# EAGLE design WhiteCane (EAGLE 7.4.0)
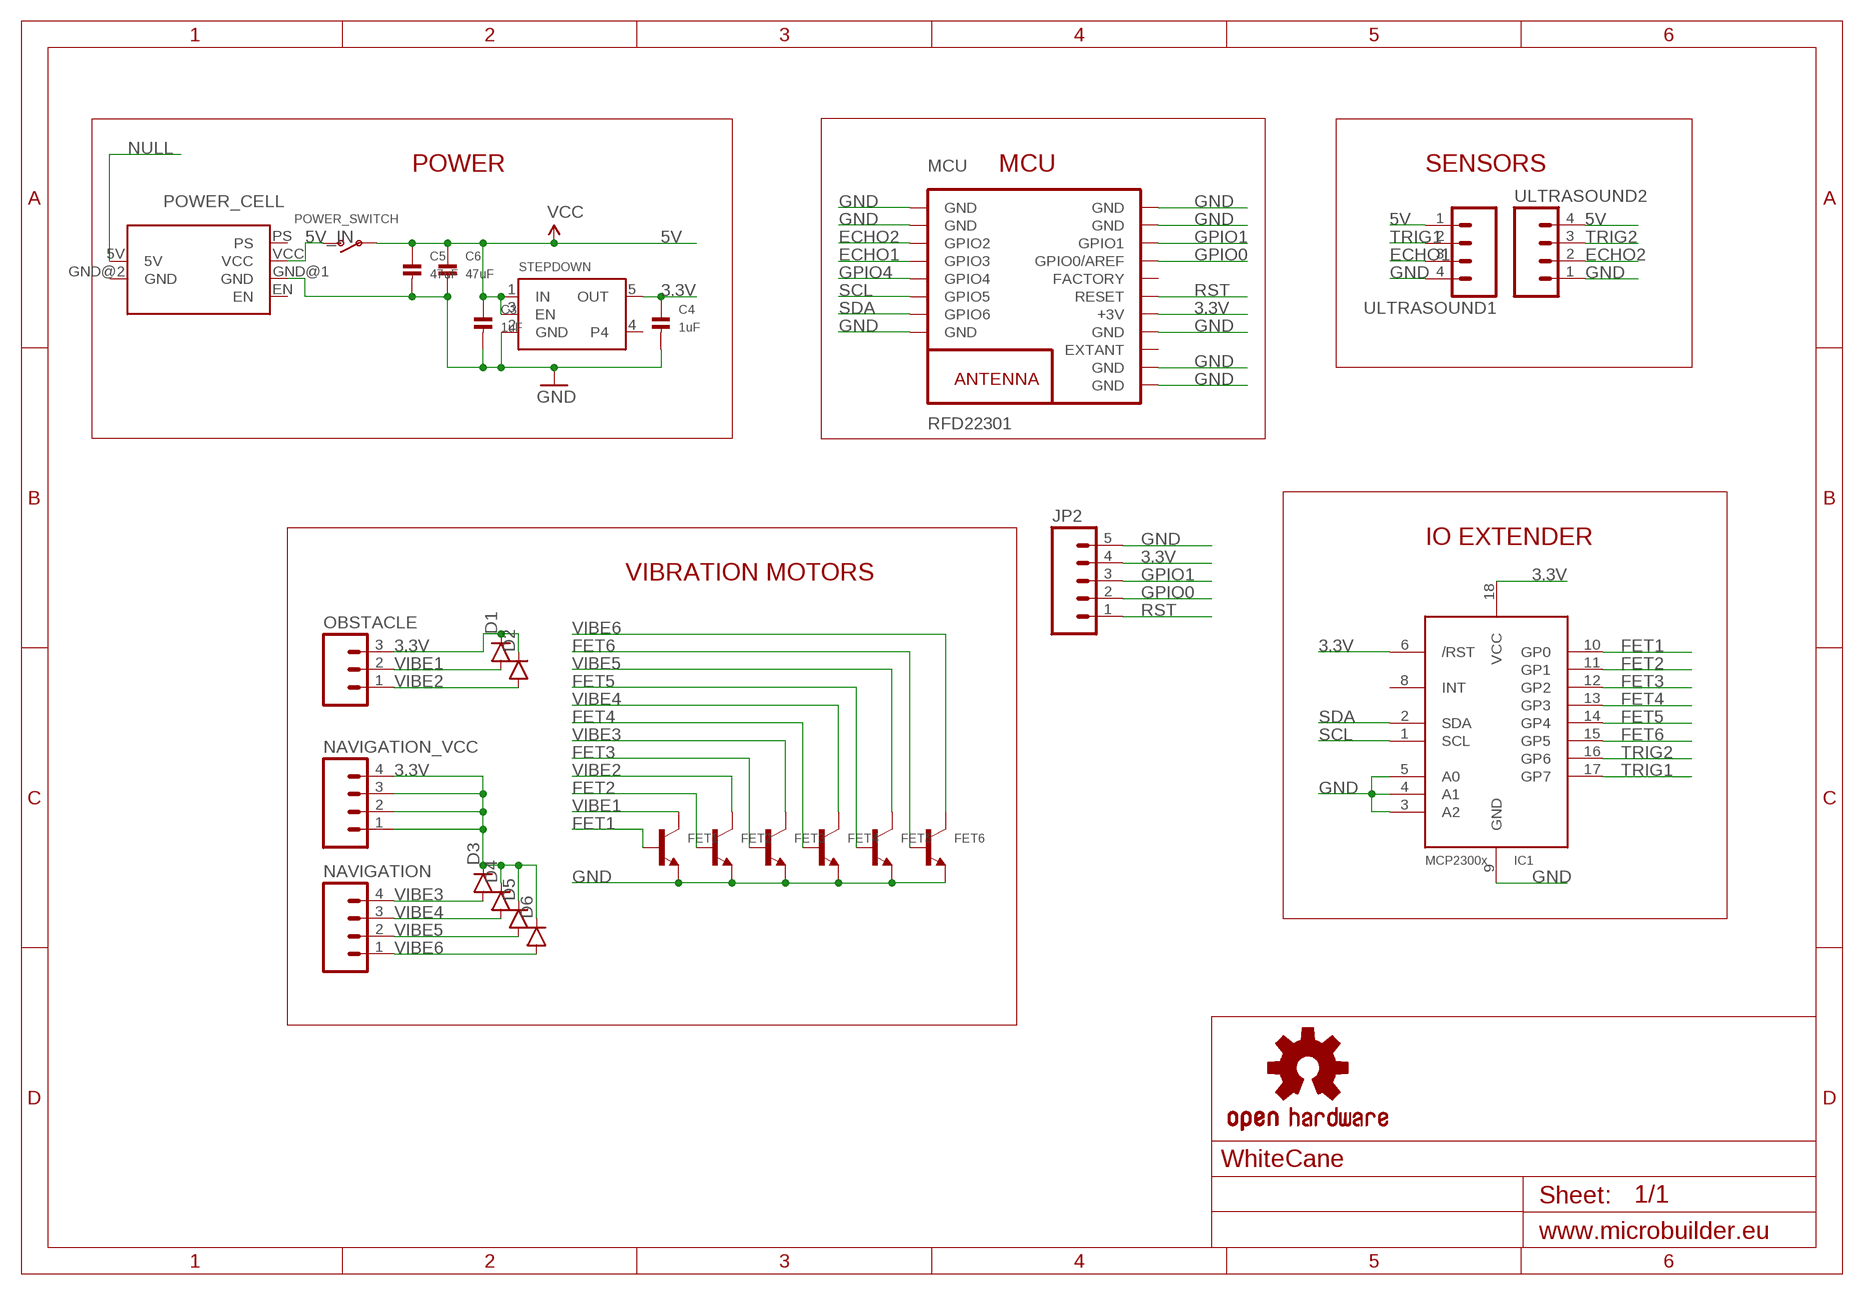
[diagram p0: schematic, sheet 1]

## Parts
C3  1uF  CAP_CERAMIC0603  [0603]
C4  1uF  CAP_CERAMIC0603  [0603]
C5  47uF  CAP_CERAMIC0805  [0805]
C6  47uF  CAP_CERAMIC0805  [0805]
D1  DIODESOD123  [SOD-123]
D2  DIODESOD123  [SOD-123]
D3  DIODESOD123  [SOD-123]
D4  DIODESOD123  [SOD-123]
D5  DIODESOD123  [SOD-123]
D6  DIODESOD123  [SOD-123]
FET1  TRANSISTOR_NPN  [SOT23-R]
FET2  TRANSISTOR_NPN  [SOT23-R]
FET3  TRANSISTOR_NPN  [SOT23-R]
FET4  TRANSISTOR_NPN  [SOT23-R]
FET5  TRANSISTOR_NPN  [SOT23-R]
FET6  TRANSISTOR_NPN  [SOT23-R]
IC1  MCP23008/SO  [SO18W]
JP2  M05PTH  [1X05]
MCU  RFD22301  [RFD22301]
NAVIGATION  M04PTH  [1X04]
NAVIGATION_VCC  M04PTH  [1X04]
OBSTACLE  M03PTH  [1X03]
POWER_CELL  POWER_CELL  [POWER_CELL]
POWER_SWITCH  SWITCH_SPST  [SPST_SMT_19192]
STEPDOWN  VREG_SOT23-5  [SOT23-5]
U$1  OSHW-LOGOS  [OSHW-LOGO-S]
ULTRASOUND1  M04PTH  [1X04]
ULTRASOUND2  M04PTH  [1X04]

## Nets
3.3V: C4.1 D1.C D2.C D3.C D4.C D5.C D6.C IC1.6(/RST) IC1.18(VCC) JP2.4 MCU.13(+3V) NAVIGATION_VCC.1 NAVIGATION_VCC.2 NAVIGATION_VCC.3 OBSTACLE.3 STEPDOWN.5(OUT)
5V: C3.1 C5.1 C6.1 POWER_SWITCH.B(P) STEPDOWN.1(IN) STEPDOWN.3(EN) ULTRASOUND1.1 ULTRASOUND2.4 ; supply symbol labelled VCC
5V_IN: POWER_CELL.VCC POWER_SWITCH.C(S)
ECHO1: MCU.4(GPIO3) ULTRASOUND1.3
ECHO2: MCU.3(GPIO2) ULTRASOUND2.2
FET1: FET1.1(B) IC1.10(GP0)
FET2: FET2.1(B) IC1.11(GP1)
FET3: FET3.1(B) IC1.12(GP2)
FET4: FET4.1(B) IC1.13(GP3)
FET5: FET5.1(B) IC1.14(GP4)
FET6: FET6.1(B) IC1.15(GP5)
GND: C3.2 C4.2 C5.2 C6.2 FET1.2(E) FET2.2(E) FET3.2(E) FET4.2(E) FET5.2(E) FET6.2(E) IC1.3(A2) IC1.4(A1) IC1.5(A0) IC1.9(GND) JP2.5 MCU.1(GND) MCU.2(GND) MCU.8(GND) MCU.9(GND) MCU.10(GND) MCU.12(GND) MCU.18(GND) MCU.19(GND) POWER_CELL.GND@1(GND) STEPDOWN.2(GND) ULTRASOUND1.4 ULTRASOUND2.1
GPIO0: JP2.2 MCU.16(GPIO0/AREF)
GPIO1: JP2.3 MCU.17(GPIO1)
GPIO4: MCU.5(GPIO4)
NULL: POWER_CELL.5V
RST: JP2.1 MCU.14(RESET)
SCL: IC1.1(SCL) MCU.6(GPIO5)
SDA: IC1.2(SDA) MCU.7(GPIO6)
TRIG1: IC1.17(GP7) ULTRASOUND1.2
TRIG2: IC1.16(GP6) ULTRASOUND2.3
VIBE1: D1.A FET1.3(C) OBSTACLE.2
VIBE2: D2.A FET2.3(C) OBSTACLE.1
VIBE3: D3.A FET3.3(C) NAVIGATION.4
VIBE4: D4.A FET4.3(C) NAVIGATION.3
VIBE5: D5.A FET5.3(C) NAVIGATION.2
VIBE6: D6.A FET6.3(C) NAVIGATION.1
Unconnected: IC1.8(INT) MCU.11(EXTANT) MCU.15(FACTORY) NAVIGATION_VCC.4 POWER_CELL.EN POWER_CELL.PS STEPDOWN.4

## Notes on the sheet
- POWER | MCU | SENSORS
- IO EXTENDER
- VIBRATION MOTORS

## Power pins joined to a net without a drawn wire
GND: POWER_CELL.GND@2(GND)

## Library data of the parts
C3-C6 = microbuilder:CAP_CERAMIC: Ceramic Capacitors
D1-D6 = SparkFun-DiscreteSemi:DIODE: Diode
FET1-FET6 = microbuilder:TRANSISTOR_NPN: NPN Transistor Transistor (NPN) 500mA 45V - BC817 [Digikey: 568-1631-1-ND] Transistor (NPN) 500mA 45V - BC817,215 [Mouser: 771-BC817-T/R] SOT23-R - SOT23 footprint optimised for use with solder paste and reflow ovens. SOT23-W - SOT23 footprint optimised for hand-soldering (larger pads).
IC1 = adafruit:MCP23008: MCP23008 Inexpensive i2c i/o expander - 8 general purpose i/o pins with optional pullups
JP2 = SparkFun-Connectors:M05: Header 5 Standard 5-pin 0.1" header. Use with straight break away headers (SKU : PRT-00116), right angle break away headers (PRT-00553), swiss pins (PRT-00743), machine pins (PRT-00117), and female headers (PRT-00115). Molex polarized connector foot print use with SKU : PRT-08230 with associated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
MCU = RF_Digital_RFD22301_Eagle_Schematic_PCB_Library:RFD22301: RFD22301 RFduino SMT Module RFD22301 Datasheet: http://www.rfdigital.com/wp-content/uploads/2014/03/RFD22301.Data_.Sheet_.11.24.13_11.38PM.pdf
NAVIGATION NAVIGATION_VCC ULTRASOUND1 ULTRASOUND2 = SparkFun-Connectors:M04: Header 4 Standard 4-pin 0.1" header. Use with straight break away headers (SKU : PRT-00116), right angle break away headers (PRT-00553), swiss pins (PRT-00743), machine pins (PRT-00117), and female headers (PRT-00115). Molex polarized connector foot print use with SKU : PRT-08231 with associated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
OBSTACLE = SparkFun-Connectors:M03: Header 3 Standard 3-pin 0.1" header. Use with straight break away headers (SKU : PRT-00116), right angle break away headers (PRT-00553), swiss pins (PRT-00743), machine pins (PRT-00117), and female headers (PRT-00115). Molex polarized connector foot print use with SKU : PRT-08232 with associated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
POWER_CELL = myParts:POWER_CELL
POWER_SWITCH = microbuilder:SWITCH_SPST: Switch - SPST
STEPDOWN = microbuilder:VREG_SOT23-5: SOT23-5 Fixed Voltage Regulators To better organise some of the SOT23-5 fixed voltage regulators in this library, this new part was created. Part Current Out V Out V In V Dropout Digikey Part No. ADP121 150mA 3.3V 3.4-5.5V 0.09V @ 150mA ADP121-AUJZ33R7CT-ND ADP121 150mA 3.0V 3.1-5.5V 0.09V @ 150mA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
U$1 = SparkFun:OSHW-LOGO: Open Source Hardware Logo This logo indicates the piece of hardware it is found on incorporates a OSHW license and/or adheres to the definition of open source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

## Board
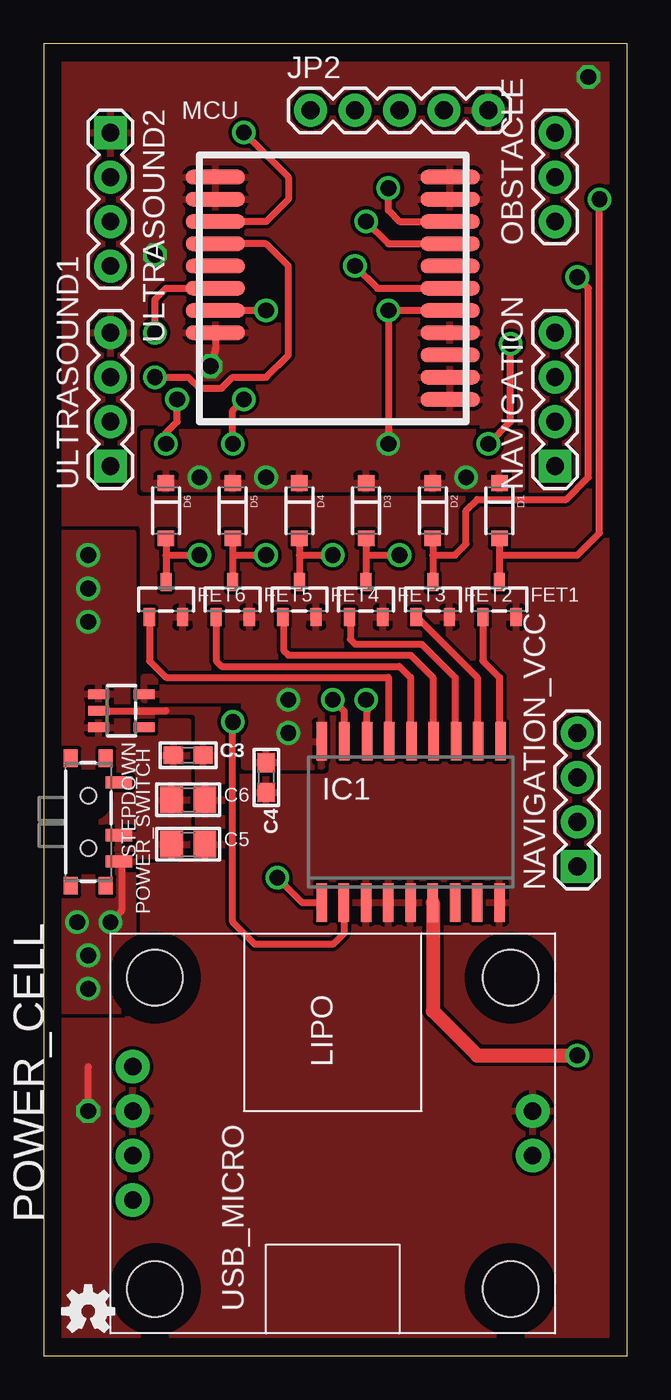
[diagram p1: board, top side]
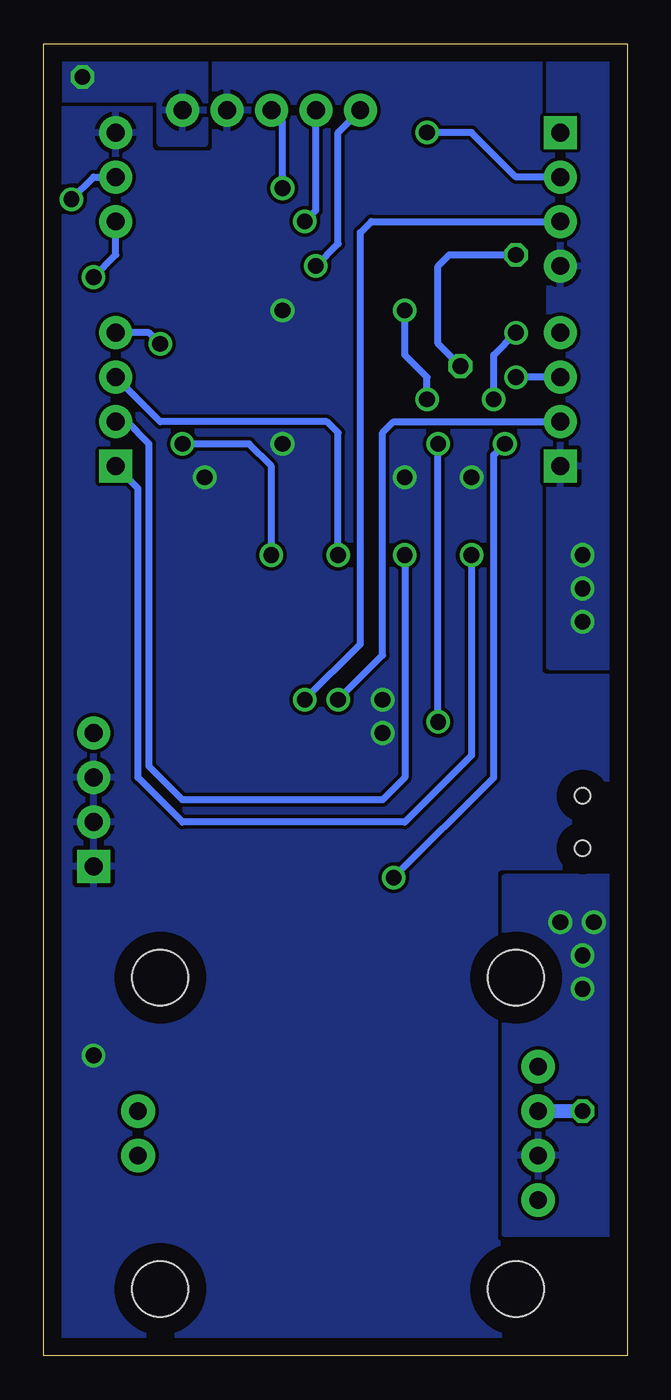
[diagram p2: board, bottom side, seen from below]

Size 33.33 x 74.92 mm. Coordinates in mm from the lower left corner, seen from the top.
Outline: 0,0 33.33,0 33.33,74.92 0,74.92 0,0
Copper layers (1*16): Top 0.035mm / dielectric 1.5mm / Bottom 0.035mm
Design rules "default": minimum track width 10mil, minimum drill 24mil, track to track 8mil, track to pad 8mil, pad to pad 8mil, via to via 8mil, smd to smd 8mil, copper to edge 40mil, drill to drill 8mil, minimum pad ring 10mil, minimum via ring 8mil, stop-mask expansion 4mil, vias tented up to drill 0mil, thermal gap 10mil

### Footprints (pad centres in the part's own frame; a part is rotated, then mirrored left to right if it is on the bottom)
0603 = smd 1.1 x 1: 1 -0.85,0; 2 0.85,0
0805 = smd 1.3 x 1.5: 1 -0.95,0; 2 0.95,0
SOD-123 = smd 0.9 x 0.95: A 1.575,0; C -1.575,0
SOT23-R = smd 0.635 x 1.016: 1 -0.95,-1; 2 0.95,-1; 3 0,1
SO18W = smd 0.6 x 2.2: 1 -4.445,-4.6; 2 -3.175,-4.6; 3 -1.905,-4.6; 4 -0.635,-4.6; 5 0.635,-4.6; 6 1.905,-4.6; 7 3.175,-4.6; 8 4.445,-4.6; 9 5.715,-4.6; 10 5.775,4.6; 11 4.505,4.6; 12 3.235,4.6; 13 1.965,4.6; 14 0.695,4.6; 15 -0.575,4.6; 16 -1.845,4.6; 17 -3.145,4.6; 18 -4.445,4.6
1X05 = drill 1.016 pad 1.88: 1 0,0; 2 2.54,0; 3 5.08,0; 4 7.62,0; 5 10.16,0
RFD22301 = smd 3.353 x 0.813: 1 -6.706,7.62; 2 -6.706,6.35; 3 -6.706,5.08; 4 -6.706,3.81; 5 -6.706,2.54; 6 -6.706,1.27; 7 -6.706,0; 8 -6.706,-1.27; 9 6.706,-5.08; 10 6.706,-3.81; 11 6.706,-2.54; 12 6.706,-1.27; 13 6.706,0; 14 6.706,1.27; 15 6.706,2.54; 16 6.706,3.81; 17 6.706,5.08; 18 6.706,6.35; 19 6.706,7.62
1X04 = drill 1.016 pad 1.88 square: 1 0,0 | drill 1.016 pad 1.88: 2 2.54,0; 3 5.08,0; 4 7.62,0
1X03 = drill 1.016 pad 1.88: 1 0,0; 2 2.54,0; 3 5.08,0
POWER_CELL = drill 1 pad 1.93: 5V -1.27,-11.43; EN 3.81,11.43; GND@1 1.27,11.43; GND@2 1.27,-11.43; PS -3.81,11.43; VCC -1.27,11.43 | hole 3.2: -8.89,10.16; 8.89,10.16; 8.89,-10.16; -8.89,-10.16
SPST_SMT_19192 = smd 0.7 x 1.5: A -2.25,1.75; B 0.75,1.75; C 2.25,1.75 | smd 1 x 0.8: GND1 -3.65,1; GND2 -3.65,-1; GND3 3.65,1; GND4 3.65,-1 | hole 0.9: -1.5,0; 1.5,0
SOT23-5 = smd 0.55 x 1.2: 1 -0.95,-1.3; 2 0,-1.3; 3 0.95,-1.3; 4 0.95,1.3; 5 -0.95,1.3

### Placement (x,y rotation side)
C3  8.25,34.29 0 top
C4  12.7,33.02 270 top
C5  8.25,29.21 0 top
C6  8.25,31.75 0 top
D1  26.04,48.26 270 top
D2  22.22,48.26 270 top
D3  18.41,48.26 270 top
D4  14.61,48.26 270 top
D5  10.79,48.26 270 top
D6  6.99,48.26 270 top
FET1  26.04,43.18 0 top
FET2  22.22,43.18 0 top
FET3  18.41,43.18 0 top
FET4  14.61,43.18 0 top
FET5  10.79,43.18 0 top
FET6  6.99,43.18 0 top
IC1  20.32,30.48 0 top
JP2  15.24,71.12 0 top
MCU  16.51,59.69 0 top
NAVIGATION  29.21,50.8 90 top
NAVIGATION_VCC  30.48,27.94 90 top
OBSTACLE  29.21,64.77 90 top
POWER_CELL  16.51,12.7 90 top
POWER_SWITCH  2.54,30.48 270 top
STEPDOWN  4.44,36.83 270 top
U$1  2.54,2.54 0 top
ULTRASOUND1  3.81,50.8 90 top
ULTRASOUND2  3.81,69.85 270 top

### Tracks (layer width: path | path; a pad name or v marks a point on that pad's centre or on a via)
3.3V  (via drill 0.9)
  Top 0.406: MCU.13 v19.68,59.69 v19.68,52.07
  Top 0.813: IC1.6 22.22,19.68 24.76,17.14 v30.48,17.14
  other vias: 8.89,50.16 12.7,50.16 24.13,50.16 13.97,37.47 13.97,35.56
  pour Bottom (rank 2): -7.62,80.01 41.91,80.01 41.91,-7.62 -7.62,-7.62
  pour Top: 5.72,52.07 5.72,49.53 27.3,49.53 27.3,52.71 5.72,52.71
  pour Top: 5.72,38.73 5.72,37.47 11.43,37.47 11.43,33.66 15.88,33.66 15.88,38.73
5V  (via drill 0.9)
  other vias: 2.54,41.91 2.54,43.82 2.54,45.72
  pour Top: 5.08,35.56 -1.27,35.56 -1.27,46.99 5.08,46.99
  pour Top: -3.81,28.57 8.25,28.57 8.25,36.2 -3.81,36.2
  pour Bottom: 4.44,39.37 -2.54,39.37 -2.54,81.28 4.44,81.28
5V_IN  (via drill 0.9)
  Top 0.406: POWER_SWITCH.C 4.44,28.07 4.44,25.4 v3.81,24.76
  other vias: 2.54,20.95 2.54,22.86 1.91,24.76
  pour Bottom: 6.99,6.98 0,6.98 0,27.3 6.99,27.3
  pour Top: 5.08,19.68 0,19.68 0,28.57 5.08,28.57
ECHO1  (via drill 0.9)
  Top 0.406: MCU.4 12.7,63.5 13.97,62.23 13.97,57.15 12.7,55.88 10.79,55.88 10.16,55.25 8.89,55.25 8.25,55.88 v6.35,55.88
  Bottom 0.406: ULTRASOUND1.3 v6.35,55.88
ECHO2  (via drill 0.9)
  Top 0.406: v11.43,69.85 13.97,67.31 13.97,66.04 12.7,64.77 MCU.3
  Bottom 0.406: ULTRASOUND2.2 6.35,67.31 8.89,69.85 v11.43,69.85
FET1
  Top 0.406: FET1.1 25.08,39.69 26.04,38.73 26.04,35.14 IC1.10
FET2
  Top 0.406: FET2.1 21.32,42.18 24.76,38.73 24.76,35.14 IC1.11
FET3
  Top 0.406: FET3.1 17.51,42.18 17.51,40.91 17.78,40.64 21.59,40.64 23.49,38.73 23.49,35.14 IC1.12
FET4
  Top 0.406: FET4.1 13.7,42.18 13.7,40.28 13.97,40.01 20.95,40.01 22.22,38.73 22.22,35.77 IC1.13
FET5
  Top 0.406: FET5.1 9.84,39.69 10.16,39.37 20.32,39.37 20.95,38.73 20.95,35.77 IC1.14
FET6
  Top 0.406: FET6.1 6.03,39.69 6.99,38.73 19.68,38.73 19.68,35.77 IC1.15
GND  (via drill 0.9)
  Top 0.406: STEPDOWN.2 6.99,36.83 | v2.54,13.97 2.54,16.51 | MCU.8 9.8,57.51 v9.52,56.52
  Bottom 0.406: v9.52,56.52 10.79,57.79 10.79,62.23 10.16,62.87 v6.35,62.87
  Bottom 0.813: POWER_CELL.GND@1 v2.54,13.97
  other vias: 31.11,73.03
  pour Top (rank 2): -2.54,76.2 35.56,76.2 35.56,-3.81 -2.54,-6.35
  pour Bottom: 24.13,74.3 24.13,69.22 26.67,69.22 26.67,71.75 32.39,71.75 32.39,74.3
GPIO0  (via drill 0.9)
  Top 0.406: v18.41,64.77 19.68,63.5 MCU.16
  Bottom 0.406: v18.41,64.77 17.78,65.41 JP2.2
GPIO1  (via drill 0.9)
  Top 0.406: MCU.17 20.32,64.77 19.68,65.41 v19.68,66.67
  Bottom 0.406: v19.68,66.67 19.68,70.48 JP2.3
RST  (via drill 0.9)
  Top 0.406: MCU.14 19.05,60.96 v17.78,62.23
  Bottom 0.406: v17.78,62.23 16.51,63.5 16.51,69.85 JP2.1
SCL  (via drill 0.9)
  Top 0.406: v6.35,58.42 6.35,60.33 6.99,60.96 MCU.6 | v6.99,52.07 6.99,52.71 7.62,53.34 v7.62,54.61 | v13.33,27.3 14.76,25.88 IC1.1
  Bottom 0.406: v13.33,27.3 7.62,33.02 7.62,51.44 v6.99,52.07 | v7.62,54.61 7.62,57.15 v6.35,58.42
SDA  (via drill 0.9)
  Top 0.406: IC1.2 17.14,24.13 16.51,23.49 12.06,23.49 10.79,24.76 v10.79,36.2 | v12.7,59.69 MCU.7 | v10.79,52.07 10.79,53.98 v11.43,54.61
  Bottom 0.406: v10.79,36.2 v10.79,52.07 | v11.43,54.61 11.43,55.88 12.7,57.15 v12.7,59.69
TRIG1  (via drill 0.9)
  Top 0.406: IC1.17 17.18,36.8 v16.51,37.47
  Bottom 0.406: v16.51,37.47 13.97,40.01 13.97,52.71 13.33,53.34 ULTRASOUND1.2
TRIG2  (via drill 0.9)
  Top 0.406: IC1.16 18.47,36.77 v18.41,37.47
  Bottom 0.406: ULTRASOUND2.3 14.61,64.77 15.24,64.14 15.24,40.64 v18.41,37.47
VIBE1  (via drill 0.9)
  Top 0.406: FET1.3 D1.A 26.04,45.72 30.48,45.72 31.75,46.99 v31.75,66.04
  Bottom 0.406: v31.75,66.04 30.48,67.31 OBSTACLE.2
VIBE2  (via drill 0.9)
  Top 0.406: 22.22,45.72 FET2.3 | D2.A 22.22,45.72 | v30.48,61.59 31.11,60.96 31.11,50.16 29.85,48.9 24.76,48.9 24.13,48.26 24.13,46.36 23.49,45.72 22.22,45.72
  Bottom 0.406: v30.48,61.59 29.21,62.87 OBSTACLE.1
VIBE3  (via drill 0.9)
  Top 0.406: FET3.3 D3.A 18.41,45.72 v20.32,45.72 | v25.4,52.07 26.67,53.34 v26.67,57.79
  Bottom 0.406: v20.32,45.72 20.32,50.8 21.59,52.07 v25.4,52.07 | v26.67,57.79 27.3,58.42 NAVIGATION.4
VIBE4  (via drill 0.9)
  Top 0.406: FET4.3 D4.A 14.61,45.72 v16.51,45.72
  Bottom 0.406: v16.51,45.72 16.51,52.71 17.14,53.34 26.67,53.34 NAVIGATION.3
VIBE5  (via drill 0.9)
  Top 0.406: FET5.3 D5.A 10.79,45.72 v12.7,45.72
  Bottom 0.406: v12.7,45.72 12.7,33.02 13.97,31.75 25.4,31.75 27.3,33.66 27.3,52.07 28.57,53.34 NAVIGATION.2
VIBE6  (via drill 0.9)
  Top 0.406: FET6.3 D6.A 6.99,45.72 v8.89,45.72
  Bottom 0.406: v8.89,45.72 8.89,34.29 12.7,30.48 25.4,30.48 27.94,33.02 27.94,49.53 NAVIGATION.1

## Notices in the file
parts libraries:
SparkFun-Connectors: Licensing: Creative Commons ShareAlike 4.0 International - https://creativecommons.org/licenses/by-sa/4.0
microbuilder: This work is placed in the public domain, and may be freely used for commercial and non-commercial work with the following conditions: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
